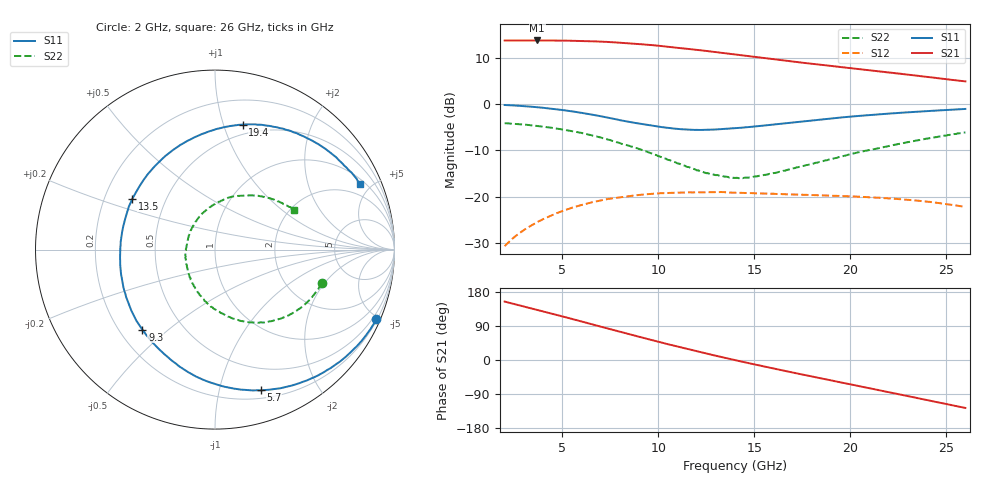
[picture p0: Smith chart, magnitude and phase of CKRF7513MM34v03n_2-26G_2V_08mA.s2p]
! CHUO DENSHI KOGYO Co.,Ltd.
! 22. July 2016
! CKRF7513MM34
! N-channel HJ-FET
! Vds = 2 V Id = 0 mA
# Hz S  MA  R 50
!	f	S11	S21	S12	S22
!	Hz	MAG	ANG	MAG	ANG	MAG	ANG	MAG	ANG
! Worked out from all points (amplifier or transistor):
!   241 points, 2 GHz to 26 GHz, reference 50 ohm
!   highest |S21| = 13.8 dB at 3.7 GHz (marker M1)
!   |S21| within 3 dB of that: start of sweep to 13.94 GHz
!   unconditionally stable (mu >= 1): 13.81 GHz to 20.94 GHz
!   at 6 GHz: K = 0.51, MSG = 17.7 dB, |S12| = -21.8 dB
!   at 14 GHz: K = 1.01, MAG = 14.4 dB, |S12| = -19.1 dB
!   at 26 GHz: K = 0.79, MSG = 13.6 dB, |S12| = -22.2 dB
!   lowest NFmin = 0.32 dB at 10 GHz
!   S11 on the Smith chart (normalised r, x): 2 GHz: 0.26, -4.83; 5.7 GHz: 0.27, -1.34; 9.3 GHz: 0.29, -0.41; 13.5 GHz: 0.32, +0.26; 19.4 GHz: 0.41, +1.16; 26 GHz: 1.26, +4.31
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2e9  0.9792 -23.3  4.878 154.2  0.02919 73.1  0.6233 -17.5
2.8e9  0.9592 -33.1  4.874 144.0  0.04059 66.6  0.606 -24.6
3.7e9  0.9257 -44.5  4.878 132.4  0.05301 59.2  0.5812 -33.0
4.7e9  0.88 -57.8  4.868 119.2  0.06622 50.8  0.5454 -42.6
5.7e9  0.8249 -72.0  4.834 105.8  0.07812 42.3  0.5018 -52.8
6e9  0.806 -76.3  4.818 101.8  0.0812 39.6  0.4891 -56.1
6.8e9  0.7534 -88.8  4.76 90.9  0.08928 32.8  0.447 -65.1
7.6e9  0.7 -102.1  4.672 79.9  0.09587 26.0  0.4011 -74.2
8.6e9  0.6369 -119.2  4.519 66.7  0.1018 18.2  0.3478 -85.8
9.3e9  0.602 -132.3  4.41 57.4  0.1059 13.0  0.3107 -95.5
1e10  0.5719 -145.9  4.283 48.2  0.1085 7.7  0.2745 -105.9
1.08e10  0.5452 -161.5  4.122 38.0  0.1102 2.0  0.2381 -117.9
1.17e10  0.5285 -179.0  3.933 26.8  0.1113 -3.8  0.2035 -134.7
1.26e10  0.5275 164.2  3.738 15.9  0.1115 -9.1  0.1793 -153.1
1.35e10  0.5408 148.4  3.549 5.3  0.1116 -14.9  0.1646 -173.7
1.4e10  0.5486 140.4  3.441 -0.3  0.1103 -17.4  0.1596 174.9
1.61e10  0.6047 111.8  3.044 -23.5  0.1071 -27.4  0.1807 131.1
1.8e10  0.6657 90.8  2.732 -43.4  0.1042 -35.5  0.2262 101.8
1.94e10  0.713 77.5  2.533 -57.9  0.102 -41.5  0.2676 85.3
2.2e10  0.7893 55.5  2.2 -84.8  0.09572 -53.5  0.3524 58.8
2.4e10  0.8427 39.2  1.972 -105.8  0.08832 -63.9  0.4237 41.6
2.6e10  0.8876 24.2  1.761 -126.5  0.0774 -74.3  0.4941 26.8
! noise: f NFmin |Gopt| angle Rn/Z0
1e+10  0.32  0.504  96.7  0.07
1.05e+10  0.34  0.48  103.8  0.07
1.1e+10  0.36  0.451  113.3  0.06
1.15e+10  0.38  0.423  122.8  0.05
1.2e+10  0.4  0.4  132.8  0.04
1.25e+10  0.42  0.38  143.8  0.04
1.3e+10  0.44  0.363  155.2  0.04
1.35e+10  0.47  0.355  167.7  0.03
1.4e+10  0.5  0.362  -179.7  0.03
1.5e+10  0.54  0.381  -159.1  0.03
